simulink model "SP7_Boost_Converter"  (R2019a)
settings: Solver=VariableStepAuto  StartTime=0  StopTime=0.02  FixedStep=1e-6  RelTol=1e-3
libraries: fl_lib x8, nesl_utility x5, ee_lib x3, powerlib_meascontrol x1

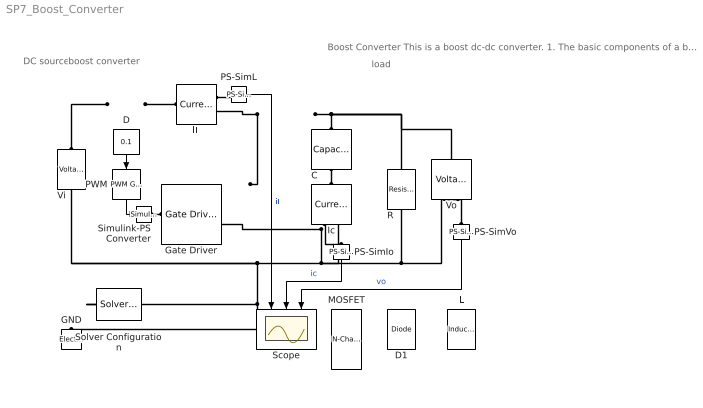
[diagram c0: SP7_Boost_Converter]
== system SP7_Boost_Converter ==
  note: Boost Converter This is a boost dc-dc converter. 1. The basic components of a boost converter are located at the bottom. 2. Place them in the appropriate positions. Press Ctrl+R to rotate a component. 3. Set the inductor value to 100 uH and output resistor to 50 Ohms. C1. Capture the complete circuit diagram. 4. Simulate the circuit. 5. Open the Scope to observe the current and voltage waveforms. C2. Capture the inductor current, capacitor current, and output voltage waveforms. Q1. Does this circuit operate in CCM, BCM, or DCM? Q2. What is the output voltage (Vo) in steady state? 6. Change the duty ratio so that the converter is in BCM. Q3. What is the duty ratio that results in BCM operation? C3. Capture the new current and voltage waveforms. Q4. What is the new output voltage (Vo) in steady state? ------------------------------------------------------- 7. Simulate duty ratios D = 0.2, 0.3, 0.4, 0.5, 0.6, 0.7, 0.8, and 0.9, and record output voltage. 8. Use Matlab to plot Vo vs. D for all simulated points, including the BCM point and D=0.1. C4. Capture the output voltage (y-axis) vs. duty ratio (x-axis) plot. 9. Use "hold on" in Matlab to overlay a trace onto the existing plot. (Look it up if you need to.) 10. Overlay a plot of Vo vs. D for CCM operation using the same D values. Q5. Describe in detail how the output voltage changes over the duty ratio range for CCM. 11. Then, o verlay a plot of Vo vs. D for DCM operation using the same D values. Q6. Describe in detail how the output voltage changes over the duty ratio range for DCM. C5. Capture the output voltage (y-axis) vs. duty ratio (x-axis) plot with all three traces. Q7. Describe the simulated points relative to the DCM and CCM curves. _________________________________ Play: Figure out how to change the switching frequency (for example, to 5 kHz). Observe how the inductor current and conduction changes at different frequencies.
  note: load
  note: DC source
  note: boost converter
  C : fl_lib/Electrical/Electrical Elements/Capacitor  c=50 uF  r=1e-6 Ohm  g=0 1/Ohm  i_specify=off  i_priority=None  i=0 A  i_nominal_specify=off  i_nominal_unit=A  i_nominal_value=1  v_specify=off  v_priority=High  v=20 V  v_nominal_specify=off  v_nominal_unit=V  v_nominal_value=1  vc_specify=off  vc_priority=High  vc=15 V  vc_nominal_specify=off  vc_nominal_unit=V  vc_nominal_value=1
  D : Constant  Value=0.1
  D1 : fl_lib/Electrical/Electrical Elements/Diode  Vf=1e-3 V  Ron=1e-3 Ohm  Goff=1e-8 1/Ohm  i_specify=off  i_priority=None  i=0 A  i_nominal_specify=off  i_nominal_unit=A  i_nominal_value=1  v_specify=off  v_priority=None  v=0 V  v_nominal_specify=off  v_nominal_unit=V  v_nominal_value=1
  GND : fl_lib/Electrical/Electrical Elements/Electrical Reference
  Gate Driver : ee_lib/Semiconductors & Converters/Gate Driver  vHigh=15 V  vLow=0 V  parameterization=1  rHigh=2 Ohm  rLow=2 Ohm  tRise=20 ns  tFall=20 ns  cLoad=10 nF  enable_faults=0  t_fault=1 s  fault_type=1  uHighValue=0.7  uLowValue=0.3  tHigh=50 ns  tLow=50 ns  ZonTime_specify=off  ZonTime_priority=None  ZonTime=0 s  ZoffTime_specify=off  ZoffTime_priority=None  ZoffTime=0 s  uHigh=2.0 V  uLow=0.8 V
  Ic : fl_lib/Electrical/Electrical Sensors/Current Sensor
  L : fl_lib/Electrical/Electrical Elements/Inductor  l=1 uH  r=0 Ohm  g=1e-9 1/Ohm  i_specify=off  i_priority=None  i=0.291 A  i_nominal_specify=off  i_nominal_unit=A  i_nominal_value=1  v_specify=off  v_priority=None  v=0 V  v_nominal_specify=off  v_nominal_unit=V  v_nominal_value=1  i_L_specify=off  i_L_priority=High  i_L=0.291 A  i_L_nominal_specify=off  i_L_nominal_unit=A  i_L_nominal_value=1
  MOSFET : ee_lib/Semiconductors & Converters/N-Channel MOSFET  parameterization=1  prmDatasheet=1  prmEquCoeff=1  Beta=5.0 A/V^2  Rds=0.025 Ohm  Id=6.0 A  Vgs=10 V  Vth=1.7 V  lam=0 1/V  Tmeas=25 degC  RS=0.0001 Ohm  RD=0.01 Ohm  C_param=1  C_GS=270 pF  C_GD=80 pF  C_DS=0 pF  C_iss=350 pF  C_rss=80 pF  C_oss=0 pF  C_GS_vec=[270, 300, 290, 280, 295, 255] pF  C_GD_vec=[450, 400, 300, 190, 95, 55] pF  C_DS_vec=[450, 410, 390, 230, 175, 115] pF  C_iss_vec=[720, 700, 590, 470, 390, 310] pF  C_rss_vec=[450, 400, 300, 190, 95, 55] pF  C_oss_vec=[900, 810, 690, 420, 270, 170] pF  C_Vds_vec=[.1, .3, 1, 3, 10, 30] V  V_GS_for_cap_data=0 V  charge_linearity_param=1  C_OX=200 pF  V_C_OX=-0.5 V  IsDiode=0 A  Vbi=0.6 V  n=1  Cj0Diode=0 pF  TT=50e-9 s  dVth_dT=-6 mV/K  Rds_T2=0.037 Ohm  Tmeas2=125 degC  BEXDatasheet=-1.5  BEXEquCoeff=-1.5  etaisDatasheet=3  etaisEquCoeff=3  TdeviceDatasheet=25 degC  TdeviceEquCoeff=25 degC  Rth=[1, 10] K/W  thermal_mass_parameterization=1  thermal_mass=[1, 1] J/K  thermal_time_constant=[1, 10] s  thermal_mass_initial_temperatures=[25, 25] degC  betaref=18 A/V^2  Vfbref=-1.1 V  gamma=3.5 V^0.50000  phib2ref=1 V  thesatref=0.4 1/V  alpha=0  Vp=5e-2 V  thesrref=0 1/V  m=8  Tref=25 degC  Cox=1500 pF  Cgso=100 pF  Cgdo=14 pF  Rsref=2e-3 Ohm  Rdref=0.17 Ohm  Rgref=8.4 Ohm  Isref=5.2e-13 A  Cj0=480 pF  Tprm=1  etabet=1.3  Stvfb=5e-4 V/K  Stphib=-8.5e-4 V/K  etasat=1.04  etasr=0.65  etar=0.95  etais=3  Tsim=25 degC  T0=[25, 25] degC
  PS-SimIo : nesl_utility/PS-Simulink Converter  PhysicalDomain=network_engine_domain  SubClassName=ps_output  LeftPortType=input  RightPortType=output  PseudoPeriodic=off  Frequencies=[]  Unit=1  AffineConversion=off
  PS-SimL : nesl_utility/PS-Simulink Converter  PhysicalDomain=network_engine_domain  SubClassName=ps_output  LeftPortType=input  RightPortType=output  PseudoPeriodic=off  Frequencies=[]  Unit=1  AffineConversion=off
  PS-SimVo : nesl_utility/PS-Simulink Converter  PhysicalDomain=network_engine_domain  SubClassName=ps_output  LeftPortType=input  RightPortType=output  PseudoPeriodic=off  Frequencies=[]  Unit=1  AffineConversion=off
  PWM : powerlib_meascontrol/Pulse & Signal Generators/PWM Generator (DC-DC)  Fsw=10000  Ts=0
  R : fl_lib/Electrical/Electrical Elements/Resistor  R=1 Ohm  i_specify=off  i_priority=None  i=0 A  i_nominal_specify=off  i_nominal_unit=A  i_nominal_value=1  v_specify=off  v_priority=None  v=0 V  v_nominal_specify=off  v_nominal_unit=V  v_nominal_value=1
  Scope : Scope  NumInputPorts=3
  Simulink-PS Converter : nesl_utility/Simulink-PS Converter  PhysicalDomain=network_engine_domain  SubClassName=ps_input  LeftPortType=input  RightPortType=output  PseudoPeriodic=off  Frequencies=[]  NoiseDistribution=none  NoiseParameters=[]  Unit=1  AffineConversion=off  FilteringAndDerivatives=provide  SimscapeFilterOrder=1  InputFilterTimeConstant=0.001  UdotUserProvided=0
  Solver Configuration : nesl_utility/Solver Configuration  PhysicalDomain=network_engine_domain  SubClassName=solver  LeftPortType=input  RightPortType=generic  Tones=[]  Harmonics=[]  SimulateNoise=off  Profile=off  UseLocalSampling=off  EnableSwitchedLinearOptims=on  FrequencyDomain=off  UseCCode=off  RelTol=0.001  AbsTol=1e-06  MinStep=1e-09  ToWorkspace=off  RevertToSquareIcSolve=off  NumHomotopyIterations=100  PhasorMode=off  PhasorModeNumHarmonics=1  DoDC=off  ResidualTolerance=1e-09  UseLocalSolver=off  LocalSolverChoice=NE_BACKWARD_EULER_ADVANCER  LocalSolverSampleTime=0.001  DoFixedCost=off  MaxNonlinIter=3  MaxModeIter=2  LinearAlgebra=auto  EquationFormulation=NE_TIME_EF  DelaysMemoryBudget=1024  AutomaticFiltering=on  FilteringTimeConstant=0.001  PartitionStorageMethod=AS_NEEDED  PartitionMemoryBudget=1024  PartitionMethod=ROBUST
  Vi : ee_lib/Sources/Voltage Source  dc_voltage=10 V  ac_voltage=0 V  ac_shift=0 rad  ac_frequency=60 Hz  noise_mode=0  PSD=0 V^2/Hz  repeatability=1  auto_seed=3646982598  user_seed=0  sample_time=1e-3 s  i_specify=off  i_priority=None  i=0 A  i_nominal_specify=off  i_nominal_unit=A  i_nominal_value=1  v_specify=off  v_priority=None  v=0 V  v_nominal_specify=off  v_nominal_unit=V  v_nominal_value=1
  Vo : fl_lib/Electrical/Electrical Sensors/Voltage Sensor
  iL : fl_lib/Electrical/Electrical Sensors/Current Sensor
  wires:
  PWM/1 -> Simulink-PS Converter/1
  D/1 -> PWM/1
  PS-SimVo/1 -> Scope/3  "vo"
  PS-SimIo/1 -> Scope/2  "ic"
  PS-SimL/1 -> Scope/1  "iL"
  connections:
  PS-SimVo/LConn1 -- Vo/RConn1
  Ic/RConn1 -- PS-SimIo/LConn1
  Gate Driver/RConn1 -- ?
  Vi/RConn1 -- Solver Configuration/RConn1 -- GND/LConn1 -- Gate Driver/RConn2 -- Vo/RConn2 -- R/RConn1 -- Ic/RConn2
  Simulink-PS Converter/RConn1 -- Gate Driver/LConn1
  iL/RConn2 -- ?
  Vi/LConn1 -- ?
  Vo/LConn1 -- R/LConn1 -- C/LConn1
  iL/LConn1 -- ?
  PS-SimL/LConn1 -- iL/RConn1
  C/RConn1 -- Ic/LConn1
